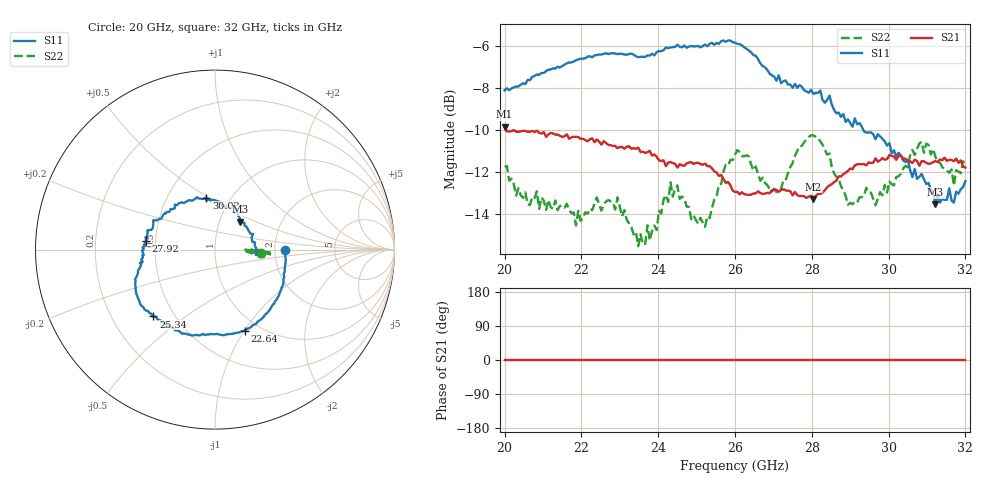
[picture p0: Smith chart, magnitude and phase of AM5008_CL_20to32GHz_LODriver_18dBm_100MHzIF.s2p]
!Keysight Technologies,N5245B,MY58422270,A.16.20.02
!Mixer S2P File: Scalar Mixer Measurement
!Calibration State: On
!Parameters: Stimulus Freq, S11, SC21, SC12, S22
# Hz  S  DB  R  50.0
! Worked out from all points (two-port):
!   201 points, 20 GHz to 32 GHz, reference 50 ohm
!   highest |S21| = -9.86 dB at 20 GHz (marker M1); lowest = -13.3 dB at 28.04 GHz (marker M2)
!   |S21| within 3 dB of the highest: start of sweep to 25.93 GHz; 28.35 GHz to end of sweep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
!   lowest |S11| = -13.5 dB at 31.22 GHz (marker M3), VSWR 1.53, Z = 62.9 + j20.4 ohm
!   |S11| at or under -10 dB: 29.34 GHz to end of sweep
!   |S22| runs from -15.5 to -10.3 dB; largest |S21 - S12| = 0.32
!   S11 on the Smith chart (normalised r, x): 20 GHz: 2.29, -0.01; 22.64 GHz: 0.85, -1.00; 25.34 GHz: 0.38, -0.38; 27.92 GHz: 0.44, +0.05; 30.02 GHz: 0.77, +0.49; 32 GHz: 1.62, -0.04
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2e10  -8.13 -0.3  -9.86 0.0  -200.00 90.0  -11.77 -4.3
2.06e10  -7.63 -21.6  -10.10 0.0  -200.00 90.0  -13.55 -2.6
2.204e10  -6.63 -58.5  -10.43 0.0  -200.00 90.0  -14.20 -3.7
2.264e10  -6.36 -70.0  -10.63 0.0  -200.00 90.0  -13.41 -2.1
2.294e10  -6.41 -76.3  -10.88 0.0  -200.00 90.0  -13.22 -2.7
2.348e10  -6.56 -88.7  -10.85 0.0  -200.00 90.0  -15.54 -0.1
2.402e10  -6.26 -100.9  -11.45 0.0  -200.00 90.0  -13.85 -2.1
2.432e10  -6.09 -107.2  -11.54 0.0  -200.00 90.0  -12.50 -3.3
2.486e10  -6.02 -121.1  -11.54 0.0  -200.00 90.0  -14.26 -2.5
2.534e10  -5.92 -132.7  -11.73 0.0  -200.00 90.0  -14.20 -1.4
2.6e10  -5.87 -146.7  -12.96 0.0  -200.00 90.0  -11.19 -3.7
2.708e10  -7.67 -170.4  -12.86 0.0  -200.00 90.0  -12.98 -2.6
2.792e10  -8.24 172.7  -13.19 0.0  -200.00 90.0  -10.35 -2.6
2.804e10  -8.29 170.6  -13.30 0.0  -200.00 90.0  -10.28 -5.1
2.894e10  -9.51 137.5  -11.96 0.0  -200.00 90.0  -13.57 -3.1
2.942e10  -10.14 122.6  -11.69 0.0  -200.00 90.0  -12.76 -3.8
2.966e10  -10.45 114.5  -11.36 0.0  -200.00 90.0  -13.59 -3.5
3.002e10  -10.63 99.3  -11.21 0.0  -200.00 90.0  -12.47 -3.6
3.086e10  -12.11 67.4  -11.50 0.0  -200.00 90.0  -10.58 -4.6
3.122e10  -13.55 47.5  -11.50 0.0  -200.00 90.0  -11.29 -4.6
3.17e10  -13.47 11.9  -11.50 0.0  -200.00 90.0  -12.66 -3.2
3.2e10  -12.45 -3.1  -11.80 0.0  -200.00 90.0  -11.82 -5.4
